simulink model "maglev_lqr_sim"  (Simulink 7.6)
settings: Solver=ode45  StartTime=0.0  StopTime=5  RelTol=1e-3
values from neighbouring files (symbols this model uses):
  C = C * 1e-5    [maglev_init.m]
  g = 9.80665    [maglev_init.m]
  L1 = L1/10    [maglev_init.m]
  m = m/100    [maglev_init.m]
  R = input('Inserire le prime due cifre (esclusi zeri) del proprio numero di matricola:\n\n')    [maglev_init.m]
  x1_0 = 0.1    [maglev_init.m]
  x1_d = 0.05    [maglev_init.m]
  x2_0 = 0    [maglev_init.m]
  x2_d = 0    [maglev_init.m]
  x3_0 = 0.2    [maglev_init.m]
undefined symbols (not defined in the file or in its folder): K, mpert
libraries: simulink x1

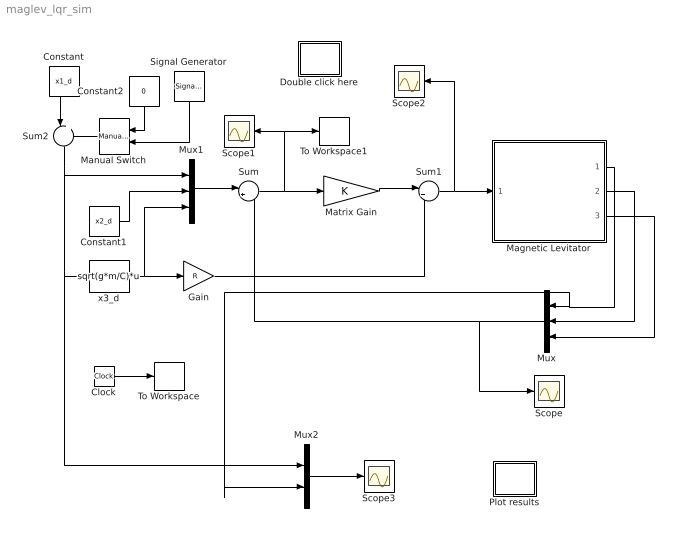
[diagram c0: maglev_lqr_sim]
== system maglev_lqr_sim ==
  Clock : Clock
  Constant : Constant  Value=x1_d
  Constant1 : Constant  Value=x2_d
  Constant2 : Constant  Value=0
  Double click here : Subsystem
  Gain : Gain  Gain=R
  Magnetic Levitator : Subsystem  mask{m=m+mpert, R=R, L1=L1, C=C, g=g}
      mask prompts: m "ball's mass (m)"; R "Electromagnet's resistance (R)"; L1 "Electromagnet's inductance (L1)"; C "Magnetic force constant (C)"; g "Gravitational acceleration (g)"
  Manual Switch : simulink/Signal Routing/Manual Switch  SystemSampleTime=-1  sw=0  action=0  varsize=off
  Matrix Gain : Gain  Gain=K  Multiplication=Matrix(K*u)
  Mux : Mux  Inputs=3
  Mux1 : Mux  Inputs=3
  Mux2 : Mux  Inputs=2
  Plot results : Subsystem
  Scope{,1..3} (4 alike) : Scope
  Signal Generator : SignalGenerator  WaveForm=square  Amplitude=x1_d*0.1  Frequency=0.5
  Sum : Sum  Inputs=|+-
  Sum1 : Sum  Inputs=|++
  Sum2 : Sum  Inputs=|++
  To Workspace : ToWorkspace  VariableName=tlq  SampleTime=-1  SaveFormat=Array
  To Workspace1 : ToWorkspace  VariableName=elq  SampleTime=-1  SaveFormat=Array
  x3_d : Fcn  Expr=sqrt(g*m/C)*u
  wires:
  x3_d/1 -> Mux1/3, Gain/1
  Constant1/1 -> Mux1/2
  Sum1/1 -> Magnetic Levitator/1(u), Scope2/1
  Sum/1 -> Matrix Gain/1, Scope1/1, To Workspace1/1
  Magnetic Levitator/1(x1) -> Mux/1, Mux2/2
  Magnetic Levitator/2(x2) -> Mux/2
  Magnetic Levitator/3(x3) -> Mux/3
  Mux/1 -> Sum/2, Scope/1
  Mux1/1 -> Sum/1
  Matrix Gain/1 -> Sum1/1
  Gain/1 -> Sum1/2
  Constant/1 -> Sum2/1
  Constant2/1 -> Manual Switch/1
  Signal Generator/1 -> Manual Switch/2
  Manual Switch/1 -> Sum2/2
  Sum2/1 -> Mux1/1, x3_d/1, Mux2/1
  Clock/1 -> To Workspace/1
  Mux2/1 -> Scope3/1

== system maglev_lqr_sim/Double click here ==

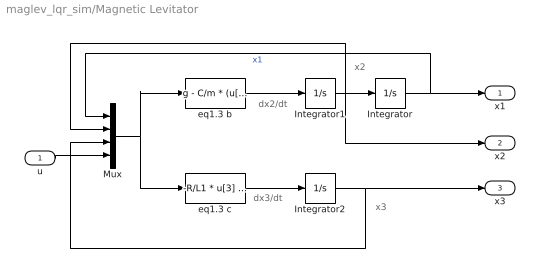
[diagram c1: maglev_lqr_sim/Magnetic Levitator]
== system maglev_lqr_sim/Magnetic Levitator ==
  note: x2
  note: x3
  note: dx2/dt
  note: dx3/dt
  u : Inport
  Integrator : Integrator  InitialCondition=x1_0
  Integrator1 : Integrator  InitialCondition=x2_0
  Integrator2 : Integrator  InitialCondition=x3_0
  Mux : Mux
  eq1.3 b : Fcn  Expr=g - C/m * (u[3] / u[1])^2
  eq1.3 c : Fcn  Expr=-R/L1 * u[3] + (2*C)/L1 * ( u[2] * u[3] / u[1]^2 ) + 1/L1 * u[4]
  x1 : Outport
  x2 : Outport  Port=2
  x3 : Outport  Port=3
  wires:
  eq1.3 b/1 -> Integrator1/1
  Integrator1/1 -> Integrator/1, Mux/2, x2/1
  eq1.3 c/1 -> Integrator2/1
  Mux/1 -> eq1.3 b/1, eq1.3 c/1
  Integrator/1 -> Mux/1, x1/1  "x1"
  Integrator2/1 -> Mux/3, x3/1
  u/1 -> Mux/4

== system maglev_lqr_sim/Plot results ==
